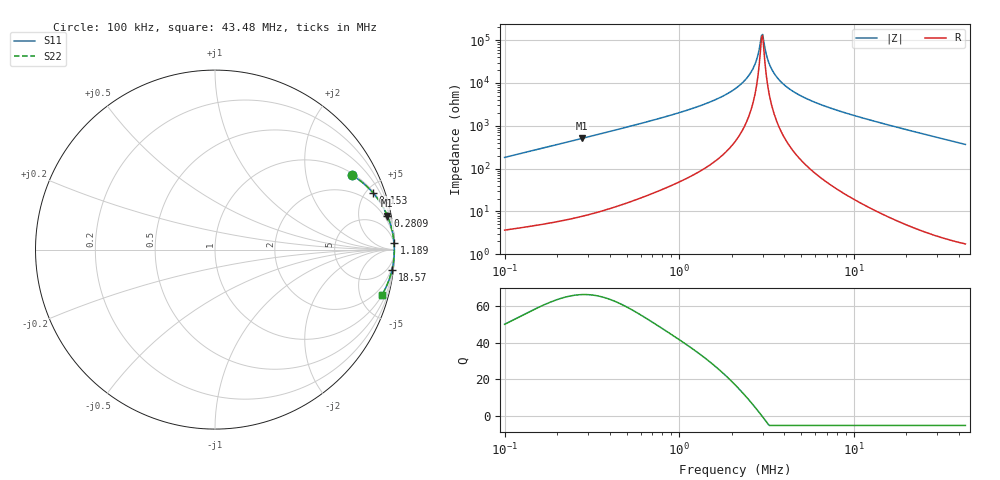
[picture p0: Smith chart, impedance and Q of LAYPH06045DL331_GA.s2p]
! LAYPH06045DL331_GA  S-PARAMETER MODEL  ( General Type )
! Model Generated by TAIYO YUDEN Corporation (http://www.ty-top.com)
! Version 2.0
! TAIYO YUDEN Control No. 180914NI43SB-FBB
! Copyright(c) 2018 TAIYO YUDEN CO.,LTD. All Rights Reserved.
! Product Description (link to TY-COMPAS)
! https://ds.yuden.co.jp/TYCOMPAS/or/detail?pn=LAYPH06045DL331MGA&u=M
! Products Name : Inductors
! Characteristics :
!  Inductance : 330 uH , SRF(min) : -Hz , DC Resistance(max) : 1.14 Ohm
!  Rated Current : Saturation :0.36 A , Temp Rise : 0.3 A (25 degC)
!  Case Size : 6.3 x 6.0 / 0.248 x 0.236 [mm/inch] , Thickness : 4.5 / 0.177 [mm/inch]
!  (Conditions: Temperature = 25 degC , DC Bias Current/Voltage = 0A / 0V)
! External Node Assignments :
!  1  o---GGG---o  2
! GND o---------o GND
! Frequency Range : 0.1MHz  -  43.477939MHz  [ 402 STEP ]
# MHz S RI R 50
! Freq[MHz].  S11 Real  S11 Imag  S21 Real  S21 Imag  S12 Real  S12 Imag  S22 Real  S22 Imag
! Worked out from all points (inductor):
!   401 points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, 100 kHz to 43.48 MHz, reference 50 ohm
!   read as one part in series: L = 289 uH near 103.1 kHz
!   highest Q = 66 at 276.6 kHz (marker M1), where L = 291 uH
!   self-resonance near 2.957 MHz
!   S11 on the Smith chart (normalised r, x): 100 kHz: 1.07, +3.65; 153 kHz: 1.09, +5.57; 280.9 kHz: 1, +10; 1.189 MHz: 2, +51; 18.57 MHz: 1, -18; 43.48 MHz: 1.03, -7.34
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0.1  0.7645 0.4144  0.2355 -0.4144  0.2355 -0.4144  0.7645 0.4144
0.152996  0.8818 0.3145  0.1182 -0.3145  0.1182 -0.3145  0.8818 0.3145
0.276637  0.9597 0.1893  0.0403 -0.1893  0.0403 -0.1893  0.9597 0.1893
0.28087  0.9608 0.1867  0.0392 -0.1867  0.0392 -0.1867  0.9608 0.1867
0.76528  0.9941 0.0673  0.00594 -0.0673  0.00594 -0.0673  0.9941 0.0673
1.188761  0.9974 0.0393  0.00262 -0.0393  0.00262 -0.0393  0.9974 0.0393
1.660349  0.9986 0.0232  0.00143 -0.0232  0.00143 -0.0232  0.9986 0.0232
2.117045  0.999 0.0131  0.000968 -0.0131  0.000968 -0.0131  0.999 0.0131
2.390537  0.9992 0.00837  0.000828 -0.00837  0.000828 -0.00837  0.9992 0.00837
2.618602  0.9992 0.00491  0.000757 -0.00491  0.000757 -0.00491  0.9992 0.00491
2.782609  0.9993 0.00262  0.000725 -0.00262  0.000725 -0.00262  0.9993 0.00262
2.912321  0.9993 0.000913  0.000708 -0.000913  0.000708 -0.000913  0.9993 0.000913
3.002138  0.9993 -0.000225  0.000701 0.000225  0.000701 0.000225  0.9993 -0.000225
3.048079  0.9993 -0.000794  0.000699 0.000794  0.000699 0.000794  0.9993 -0.000794
3.190166  0.9993 -0.0025  0.000696 0.0025  0.000696 0.0025  0.9993 -0.0025
3.288551  0.9993 -0.00365  0.000697 0.00365  0.000697 0.00365  0.9993 -0.00365
3.657416  0.9993 -0.00768  0.000726 0.00768  0.000726 0.00768  0.9993 -0.00768
4.388564  0.9991 -0.0148  0.000866 0.0148  0.000866 0.0148  0.9991 -0.0148
5.768256  0.9987 -0.0265  0.00133 0.0265  0.00133 0.0265  0.9987 -0.0265
15.95712  0.99 -0.096  0.00998 0.096  0.00998 0.096  0.99 -0.096
18.57425  0.9865 -0.1124  0.0135 0.1124  0.0135 0.1124  0.9865 -0.1124
43.47794  0.9298 -0.2531  0.0702 0.2531  0.0702 0.2531  0.9298 -0.2531
